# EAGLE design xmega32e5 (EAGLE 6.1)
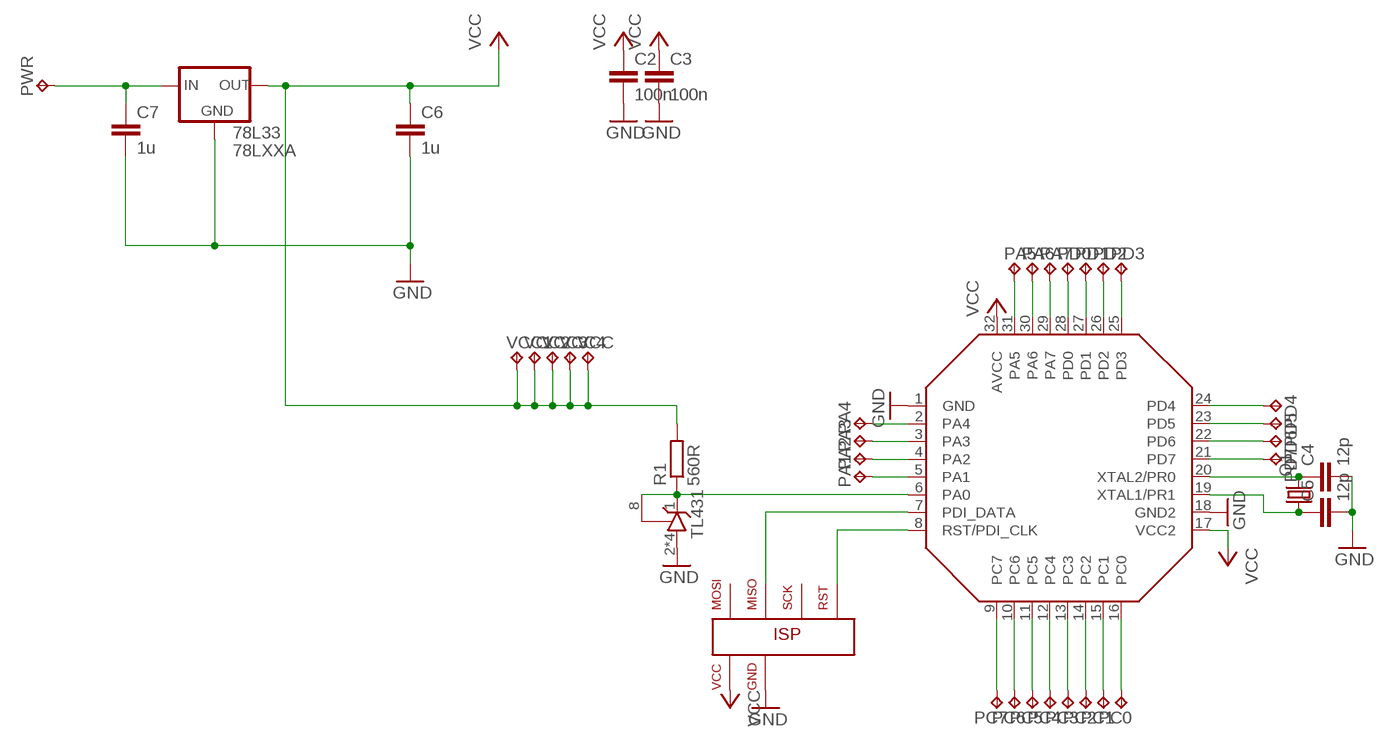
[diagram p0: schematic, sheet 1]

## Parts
78L33  78LXXA  [SO8]
ATXMEGA32E5  ATXMEGA32E5  [VQFP32]
C2  100n  C-EUC0603  [C0603]
C3  100n  C-EUC0603  [C0603]
C4  12p  C-EUC0603  [C0603]
C5  12p  C-EUC0603  [C0603]
C6  1u  C-EUC0603  [C0603]
C7  1u  C-EUC0603  [C0603]
PA1  TPTP20SQ  [TP20SQ]
PA2  TPTP20SQ  [TP20SQ]
PA3  TPTP20SQ  [TP20SQ]
PA4  TPTP20SQ  [TP20SQ]
PA5  TPTP20SQ  [TP20SQ]
PA6  TPTP20SQ  [TP20SQ]
PA7  TPTP20SQ  [TP20SQ]
PC0  TPTP20SQ  [TP20SQ]
PC1  TPTP20SQ  [TP20SQ]
PC2  TPTP20SQ  [TP20SQ]
PC3  TPTP20SQ  [TP20SQ]
PC4  TPTP20SQ  [TP20SQ]
PC5  TPTP20SQ  [TP20SQ]
PC6  TPTP20SQ  [TP20SQ]
PC7  TPTP20SQ  [TP20SQ]
PD0  TPTP20SQ  [TP20SQ]
PD1  TPTP20SQ  [TP20SQ]
PD2  TPTP20SQ  [TP20SQ]
PD3  TPTP20SQ  [TP20SQ]
PD4  TPTP20SQ  [TP20SQ]
PD5  TPTP20SQ  [TP20SQ]
PD6  TPTP20SQ  [TP20SQ]
PD7  TPTP20SQ  [TP20SQ]
PDI  ISPSMALL  [MLW06G]
PWR  TPTP20SQ  [TP20SQ]
Q1  CRYSTALHC49S  [HC49/S]
R1  560R  R-EU_R0805  [R0805]
TL431  TL431CLP  [SO8]
VCC  TPTP20SQ  [TP20SQ]
VCC1  TPTP20SQ  [TP20SQ]
VCC2  TPTP20SQ  [TP20SQ]
VCC3  TPTP20SQ  [TP20SQ]
VCC4  TPTP20SQ  [TP20SQ]

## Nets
GND: 78L33.2(GND) 78L33.3(GND) 78L33.6(GND) 78L33.7(GND) ATXMEGA32E5.1(GND) ATXMEGA32E5.18(GND2) C2.2 C3.2 C4.2 C5.2 C6.2 C7.2 PDI.6(GND) TL431.2(A) TL431.3(A) TL431.6(A) TL431.7(A)
N$1: ATXMEGA32E5.6(PA0) R1.1 TL431.1(C) TL431.8(R)
N$2: ATXMEGA32E5.20(XTAL2/PR0) C4.1 Q1.2
N$3: ATXMEGA32E5.19(XTAL1/PR1) C5.1 Q1.1
N$4: ATXMEGA32E5.16(PC0) PC0.TP
N$5: ATXMEGA32E5.8(RST/PDI_CLK) PDI.5(RST)
N$6: ATXMEGA32E5.7(PDI_DATA) PDI.1(MISO)
N$7: ATXMEGA32E5.15(PC1) PC1.TP
N$8: ATXMEGA32E5.14(PC2) PC2.TP
N$9: ATXMEGA32E5.13(PC3) PC3.TP
N$10: ATXMEGA32E5.12(PC4) PC4.TP
N$11: ATXMEGA32E5.11(PC5) PC5.TP
N$12: ATXMEGA32E5.10(PC6) PC6.TP
N$13: ATXMEGA32E5.9(PC7) PC7.TP
N$14: ATXMEGA32E5.28(PD0) PD0.TP
N$15: ATXMEGA32E5.27(PD1) PD1.TP
N$16: ATXMEGA32E5.26(PD2) PD2.TP
N$17: ATXMEGA32E5.25(PD3) PD3.TP
N$18: ATXMEGA32E5.24(PD4) PD4.TP
N$19: ATXMEGA32E5.23(PD5) PD5.TP
N$20: ATXMEGA32E5.22(PD6) PD6.TP
N$21: ATXMEGA32E5.21(PD7) PD7.TP
N$23: 78L33.8(IN) C7.1 PWR.TP
N$26: ATXMEGA32E5.5(PA1) PA1.TP
N$27: ATXMEGA32E5.4(PA2) PA2.TP
N$28: ATXMEGA32E5.3(PA3) PA3.TP
N$29: ATXMEGA32E5.2(PA4) PA4.TP
N$30: ATXMEGA32E5.31(PA5) PA5.TP
N$31: ATXMEGA32E5.30(PA6) PA6.TP
N$32: ATXMEGA32E5.29(PA7) PA7.TP
VCC: 78L33.1(OUT) ATXMEGA32E5.17(VCC2) ATXMEGA32E5.32(AVCC) C2.1 C3.1 C6.1 PDI.2(VCC) R1.2 VCC1.TP VCC2.TP VCC3.TP VCC4.TP VCC.TP
Unconnected: PDI.3(SCK) PDI.4(MOSI)

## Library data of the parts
78L33 = v-reg:78LXXA
ATXMEGA32E5 = atmel:ATXMEGA32E5: 8/16-bit Atmel AVR XMEGA Microcontrollers
C2-C7 = rcl:C-EU: CAPACITOR, European symbol
PA1-PA7 PC0 PC1-PC7 PD0 PD1-PD7 PWR VCC VCC1-VCC4 = testpad:TP: Test pad
PDI = PaJa_konektory:ISP
Q1 = crystal:CRYSTAL: CRYSTAL; OC_FARNELL: 1667008; OC_NEWARK: unknown
R1 = rcl:R-EU_: RESISTOR, European symbol
TL431 = v-reg:TL431CLP: VOLTAGE REGULATOR

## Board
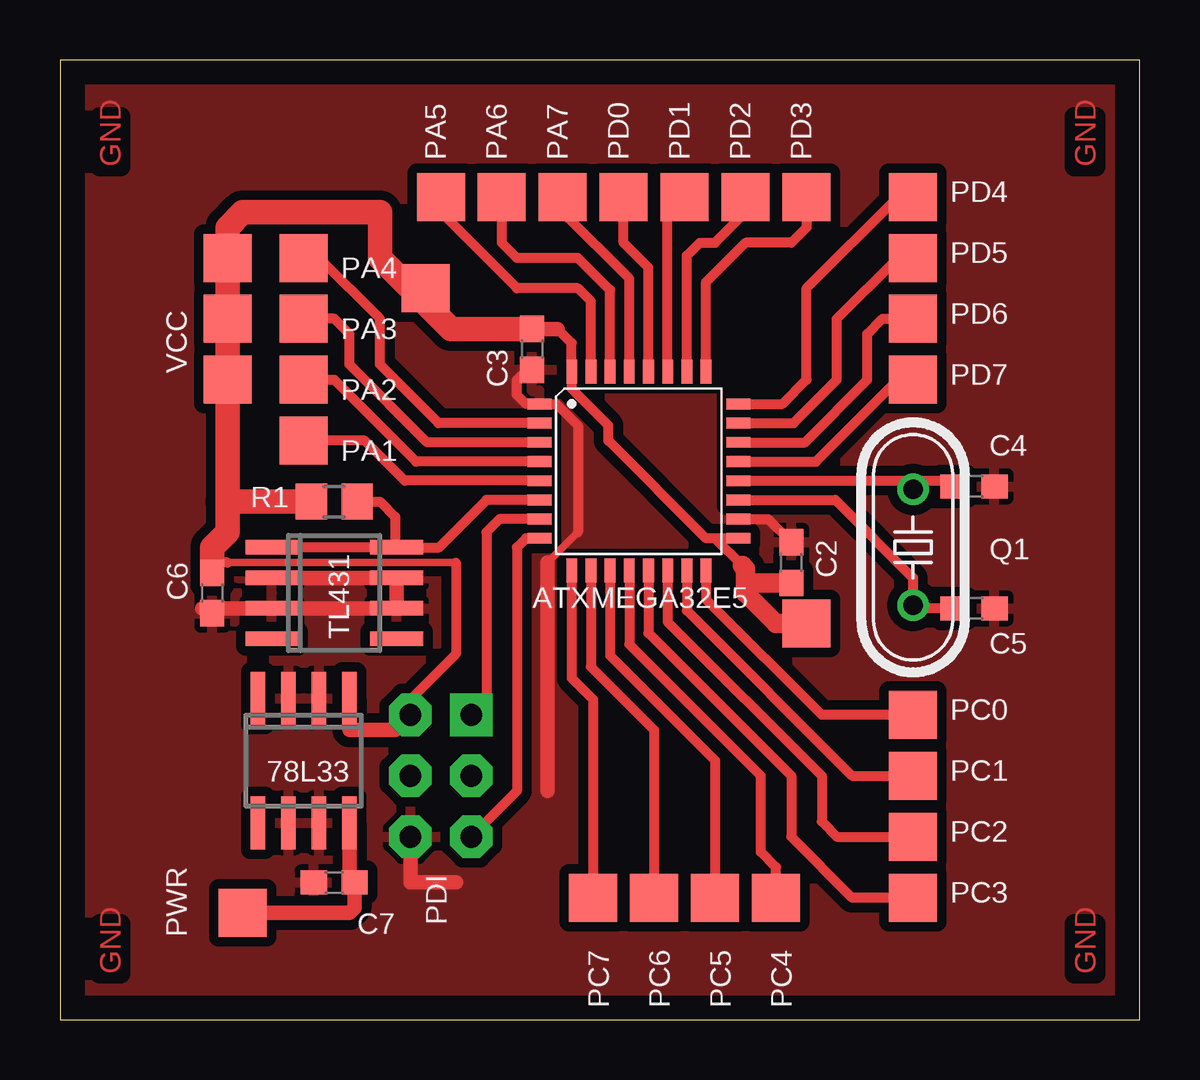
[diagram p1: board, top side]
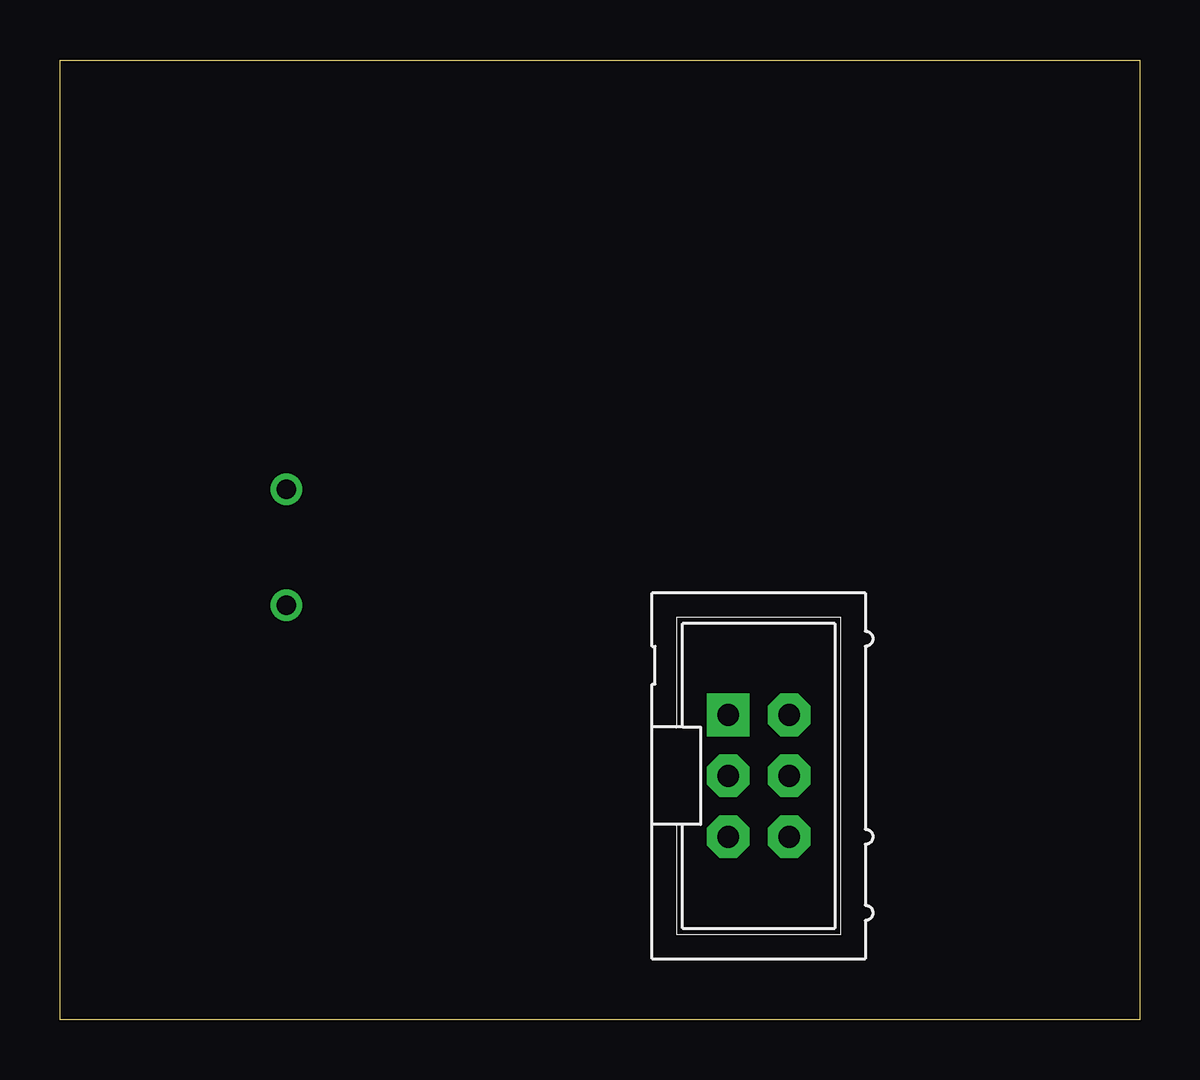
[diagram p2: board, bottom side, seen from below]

Size 45 x 40 mm. Coordinates in mm from the lower left corner, seen from the top.
Outline: 0,0 45,0 45,40 0,40 0,0
Copper layers (1*16): Top 0.035mm / dielectric 1.5mm / Bottom 0.035mm
Design rules: minimum track width 10mil, minimum drill 24mil, track to track 8mil, track to pad 8mil, pad to pad 8mil, via to via 8mil, smd to smd 8mil, copper to edge 40mil, drill to drill 8mil, minimum pad ring 10mil, minimum via ring 8mil, stop-mask expansion 4mil, vias tented up to drill 0mil, thermal gap 10mil

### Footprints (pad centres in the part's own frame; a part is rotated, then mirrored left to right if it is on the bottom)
SO8 = smd 0.6 x 2.2: 1 -1.905,-2.6; 2 -0.635,-2.6; 3 0.635,-2.6; 4 1.905,-2.6; 5 1.905,2.6; 6 0.635,2.6; 7 -0.635,2.6; 8 -1.905,2.6
VQFP32 = smd 1 x 0.45: 1 -4.15,2.8; 2 -4.15,2; 3 -4.15,1.2; 4 -4.15,0.4; 5 -4.15,-0.4; 6 -4.15,-1.2; 7 -4.15,-2; 8 -4.15,-2.8; 17 4.15,-2.8; 18 4.15,-2; 19 4.15,-1.2; 20 4.15,-0.4; 21 4.15,0.4; 22 4.15,1.2; 23 4.15,2; 24 4.15,2.8 | smd 0.45 x 1: 9 -2.8,-4.15; 10 -2,-4.15; 11 -1.2,-4.15; 12 -0.4,-4.15; 13 0.4,-4.15; 14 1.2,-4.15; 15 2,-4.15; 16 2.8,-4.15; 25 2.8,4.15; 26 2,4.15; 27 1.2,4.15; 28 0.4,4.15; 29 -0.4,4.15; 30 -1.2,4.15; 31 -2,4.15; 32 -2.8,4.15
C0603 = smd 1.1 x 1: 1 -0.85,0; 2 0.85,0
TP20SQ = smd 2 x 2: TP 0,0
MLW06G = drill 0.914 pad 1.778 square: 1 -2.54,-1.27 | drill 0.914 pad 1.778 octagon: 2 -2.54,1.27; 3 0,-1.27; 4 0,1.27; 5 2.54,-1.27; 6 2.54,1.27
HC49/S = drill 0.813: 1 -2.413,0; 2 2.413,0
R0805 = smd 1.3 x 1.5: 1 -0.95,0; 2 0.95,0

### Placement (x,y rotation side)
78L33  10.16,10.79 180 top
ATXMEGA32E5  24.13,22.86 0 top
C2  30.48,19.05 90 top
C3  19.68,27.94 270 top
C4  38.1,22.23 0 top
C5  38.1,17.14 0 top
C6  6.35,17.78 270 top
C7  11.43,5.71 180 top
PA1  10.16,24.13 0 top
PA2  10.16,26.67 0 top
PA3  10.16,29.21 0 top
PA4  10.16,31.75 0 top
PA5  15.88,34.29 0 top
PA6  18.41,34.29 0 top
PA7  20.95,34.29 0 top
PC0  35.56,12.7 0 top
PC1  35.56,10.16 0 top
PC2  35.56,7.62 0 top
PC3  35.56,5.08 0 top
PC4  29.84,5.08 0 top
PC5  27.3,5.08 0 top
PC6  24.77,5.08 0 top
PC7  22.23,5.08 0 top
PD0  23.5,34.29 0 top
PD1  26.04,34.29 0 top
PD2  28.57,34.29 0 top
PD3  31.11,34.29 0 top
PD4  35.56,34.29 0 top
PD5  35.56,31.75 0 top
PD6  35.56,29.21 0 top
PD7  35.56,26.67 0 top
PDI  15.88,10.16 270 bottom
PWR  7.62,4.45 0 top
Q1  35.56,19.68 90 top
R1  11.43,21.59 180 top
TL431  11.43,17.78 270 top
VCC  31.11,16.51 0 top
VCC1  6.99,26.67 0 top
VCC2  6.99,29.21 0 top
VCC3  6.99,31.75 0 top
VCC4  15.24,30.48 0 top

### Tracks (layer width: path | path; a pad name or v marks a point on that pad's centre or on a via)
GND
  Top 0.305: 21.59,20.32 20.32,19.05
  Top 0.406: 21.59,20.32 21.59,24.77 20.7,25.66 ATXMEGA32E5.1 19.43,25.66 19.05,26.04 19.05,26.67 19.47,27.09 C3.2 | ATXMEGA32E5.18 29.52,20.86 C2.2
  Top 0.61: 5.93,17.14 TL431.3 TL431.6 TL431.7 TL431.2 | 20.32,19.05 20.32,9.53 | 16.51,5.71 14.61,5.71 PDI.6
  pour Top (isolate 0.406): 0,40 45,40 45,0 0,0
N$1
  Top 0.406: ATXMEGA32E5.6 17.78,21.66 15.8,19.68 TL431.8 | TL431.8 TL431.1 | R1.1 13.34,21.59 13.97,20.95 13.97,19.75 TL431.8
N$2
  Top 0.406: ATXMEGA32E5.20 35.56,22.46 | 35.56,22.46 37.02,22.46 C4.1 | Q1.2 35.56,22.46
N$3
  Top 0.406: ATXMEGA32E5.19 32.31,21.66 35.56,18.41 Q1.1 35.69,17.14 C5.1
N$4
  Top 0.406: ATXMEGA32E5.16 26.93,17.52 31.75,12.7 PC0.TP
N$5
  Top 0.406: ATXMEGA32E5.8 19.43,20.06 19.05,19.68 19.05,9.53 PDI.5
N$6
  Top 0.406: ATXMEGA32E5.7 18.32,20.86 17.78,20.32 17.78,13.34 PDI.1
N$7
  Top 0.406: ATXMEGA32E5.15 26.13,17.05 33.02,10.16 PC1.TP 34.92,10.16
N$8
  Top 0.406: ATXMEGA32E5.14 25.33,16.58 31.75,10.16 31.75,8.26 32.38,7.62 PC2.TP
N$9
  Top 0.406: ATXMEGA32E5.13 24.53,16.11 30.48,10.16 30.48,7.62 33.02,5.08 PC3.TP
N$10
  Top 0.406: ATXMEGA32E5.12 23.73,15.64 29.21,10.16 29.21,6.99 29.84,6.35 PC4.TP
N$11
  Top 0.406: ATXMEGA32E5.11 22.93,15.17 27.3,10.79 PC5.TP
N$12
  Top 0.406: ATXMEGA32E5.10 22.13,14.7 24.77,12.06 PC6.TP
N$13
  Top 0.406: ATXMEGA32E5.9 21.33,14.23 22.23,13.34 PC7.TP
N$14
  Top 0.406: ATXMEGA32E5.28 24.53,31.35 23.5,32.38 PD0.TP
N$15
  Top 0.406: ATXMEGA32E5.27 25.33,33.59 PD1.TP
N$16
  Top 0.406: ATXMEGA32E5.26 26.13,31.84 26.67,32.38 27.3,32.38 28.57,33.66 PD2.TP
N$17
  Top 0.406: ATXMEGA32E5.25 26.93,30.74 28.57,32.38 30.48,32.38 31.11,33.02 PD3.TP
N$18
  Top 0.406: ATXMEGA32E5.24 30.11,25.66 31.11,26.67 31.11,30.48 34.92,34.29 PD4.TP
N$19
  Top 0.406: ATXMEGA32E5.23 30.57,24.86 32.38,26.67 32.38,29.21 34.92,31.75 PD5.TP
N$20
  Top 0.406: ATXMEGA32E5.22 31.05,24.06 33.66,26.67 33.66,28.57 34.29,29.21 PD6.TP 34.92,29.21
N$21
  Top 0.406: ATXMEGA32E5.21 31.52,23.26 34.92,26.67 PD7.TP
N$23
  Top 0.61: 78L33.8 12.06,5.93 C7.1 12.28,4.66 12.06,4.45 PWR.TP
N$26
  Top 0.406: ATXMEGA32E5.5 14.37,22.46 12.7,24.13 PA1.TP
N$27
  Top 0.406: ATXMEGA32E5.4 14.84,23.26 11.43,26.67 PA2.TP
N$28
  Top 0.406: ATXMEGA32E5.3 15.31,24.06 12.06,27.3 12.06,28.57 11.43,29.21 PA3.TP
N$29
  Top 0.406: ATXMEGA32E5.2 15.78,24.86 13.34,27.3 13.34,29.21 10.79,31.75 PA4.TP
N$30
  Top 0.406: ATXMEGA32E5.31 22.13,29.94 21.59,30.48 19.05,30.48 15.88,33.66 PA5.TP
N$31
  Top 0.406: ATXMEGA32E5.30 22.93,30.41 21.59,31.75 19.05,31.75 18.41,32.38 PA6.TP
N$32
  Top 0.406: ATXMEGA32E5.29 23.73,30.88 20.95,33.66 PA7.TP
VCC
  Top 0.305: 6.99,19.05 16.51,19.05
  Top 0.406: ATXMEGA32E5.17 27.3,20.06 | 27.3,20.06 26.93,20.06 22.86,24.13 22.86,24.77 21.33,26.3 ATXMEGA32E5.32 21.33,28.2 20.74,28.79 | 28.45,18.92 27.3,20.06 | 16.51,19.05 16.51,15.24 14.61,13.34 PDI.2 | 6.99,19.05 6.77,19.05 C6.1
  Top 0.61: C3.1 20.74,28.79 | 78L33.1 12.06,12.06 13.97,12.06 PDI.2
  Top 0.813: VCC.TP 29.84,16.51 28.57,17.78 28.57,18.41 | 28.57,18.41 28.57,18.79 28.45,18.92 | C2.1 28.79,18.2 28.57,18.41
  Top 1.016: 6.99,21.59 VCC1.TP VCC2.TP VCC3.TP 6.99,33.02 7.62,33.66 13.34,33.66 13.34,31.75 15.24,29.84 | 6.99,21.59 6.99,20.32 6.35,19.68 C6.1 | C3.1 16.3,28.79 15.24,29.84 | VCC4.TP 15.24,29.84 | R1.2 6.99,21.59

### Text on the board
Top: GND | GND | GND | GND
